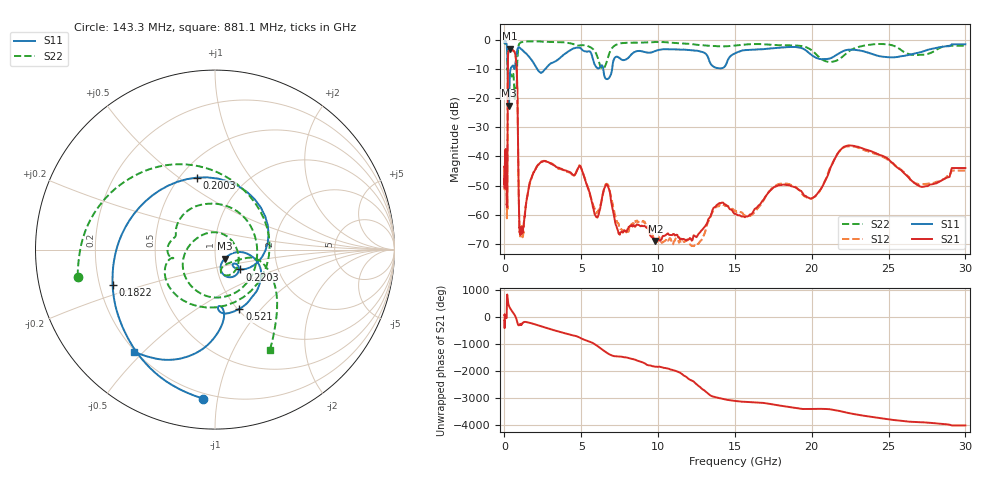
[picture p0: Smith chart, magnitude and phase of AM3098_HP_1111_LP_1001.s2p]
! Date/Time: Thu, Feb 28, 2019 8:47 AM
! Network Analyzer: Agilent Technologies E8364B Rev: A.07.50.67
! Sweep from 0.010 to 30.000 GHz, 1601 Points, Sweep Type: LOG
! Power Supply: 5.022 V, 0.002 A
# Hz S DB R 50
!freq MagS11 AngS11 MagS21 AngS21 MagS12 AngS12 MagS22 AngS22
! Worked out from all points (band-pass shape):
!   1601 points, 10 MHz to 30 GHz, reference 50 ohm
!   highest |S21| = -3.06 dB at 335.4 MHz (marker M1); lowest = -69.0 dB at 9.829 GHz (marker M2)
!   |S21| within 3 dB of the highest: 228.4 MHz to 737.2 MHz (508.8 MHz wide, 105 % of centre)
!   lowest |S11| = -22.6 dB at 293 MHz (marker M3), VSWR 1.16, Z = 55.5 - j5.57 ohm
!   |S11| at or under -10 dB: 210.1 MHz to 398.5 MHz (188.4 MHz wide, 61.9 % of centre); 2.12 GHz to 2.667 GHz (546.9 MHz wide, 22.8 % of centre); 6.429 GHz to 7.006 GHz (577.2 MHz wide, 8.59 % of centre)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
!   |S22| runs from -20.3 to -0.5 dB; largest |S21 - S12| = 0.0087
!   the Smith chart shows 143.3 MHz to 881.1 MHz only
!   S11 on the Smith chart (normalised r, x): 143.3 MHz: 0.17, -0.91; 182.2 MHz: 0.25, -0.16; 200.3 MHz: 0.61, +0.59; 220.3 MHz: 1.29, -0.29; 521 MHz: 1.02, -0.77; 881.1 MHz: 0.20, -0.47
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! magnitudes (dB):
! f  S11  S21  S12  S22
! 10 MHz  -0.4  -43.8  -45.3  -0.6
! 38.04 MHz  -0.2  -41.0  -40.8  -0.7
! 93.63 MHz  -0.8  -38.3  -38.3  -1.4
! 143.3 MHz  -1.6  -54.4  -54.7  -2.2
! 144.7 MHz  -1.6  -54.9  -55.0  -2.2
! 182.2 MHz  -4.4  -57.0  -57.9  -5.8
! 200.3 MHz  -7.7  -32.8  -32.5  -10.4
! 220.3 MHz  -15.0  -8.5  -8.5  -10.6
! 293 MHz  -22.6  -3.3  -3.2  -12.5
! 335.4 MHz  -13.6  -3.1  -3.0  -12.2
! 521 MHz  -8.9  -3.5  -3.5  -11.8
! 550.5 MHz  -8.8  -3.7  -3.6  -11.4
! 777.5 MHz  -5.6  -8.5  -8.5  -18.8
! 881.1 MHz  -2.8  -33.5  -33.5  -3.9
! 1.019 GHz  -2.9  -66.4  -67.3  -1.1
! 2.084 GHz  -9.6  -43.8  -43.7  -0.6
! 4.927 GHz  -2.8  -43.3  -43.2  -1.9
! 7.926 GHz  -6.7  -65.8  -66.0  -1.0
! 9.829 GHz  -3.8  -69.0  -68.7  -0.8
! 20 GHz  -5.3  -54.4  -54.4  -3.6
! 22.56 GHz  -3.4  -36.2  -36.5  -3.5
! 30 GHz  -1.6  -44.0  -44.8  -2.1
